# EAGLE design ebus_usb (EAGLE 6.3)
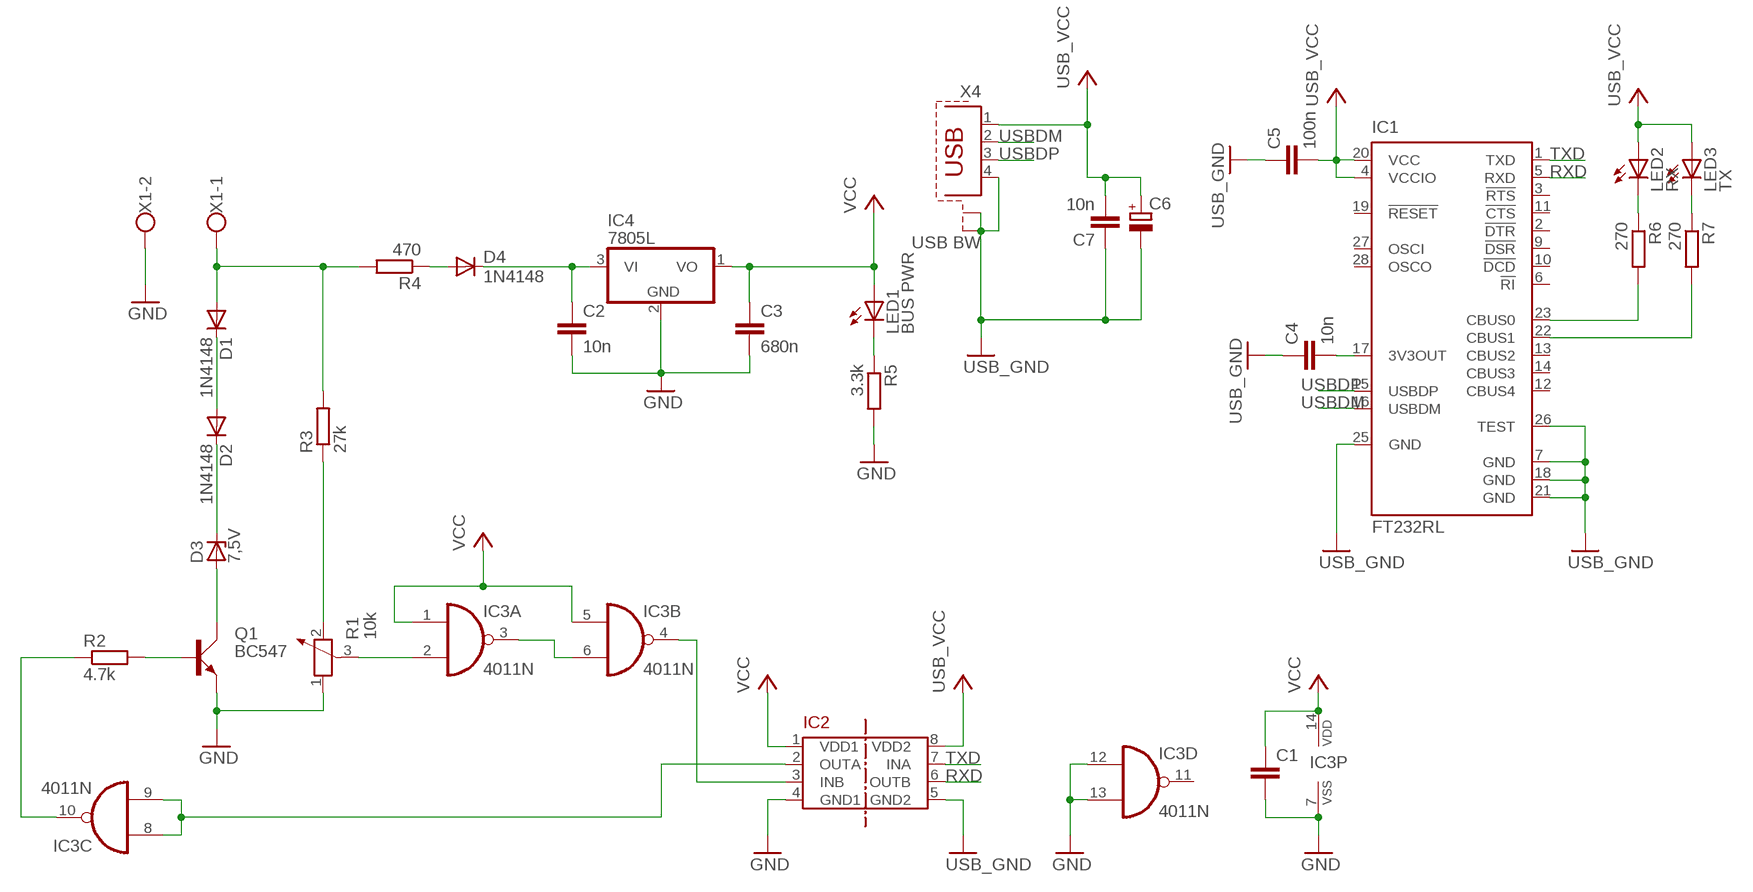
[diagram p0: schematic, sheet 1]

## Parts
C1  C-EUC0805  [C0805]
C2  10n  C-EUC0805  [C0805]
C3  680n  C-EU050-045X075  [C050-045X075]
C4  10n  C-EUC0805  [C0805]
C5  100n  C-EUC0805  [C0805]
C6  CPOL-EUE2.5-6  [E2,5-6]
C7  10n  C-EUC0805  [C0805]
D1  1N4148  1N4148DO35-7  [DO35-7]
D2  1N4148  1N4148DO35-7  [DO35-7]
D3  7,5V  ZENER-DIODEDO34-7  [DO34Z7]
D4  1N4148  1N4148DO35-7  [DO35-7]
IC1  FT232RL  [SSOP28]
IC2  ADUM1201  [SO8]
IC3  4011N  [DIL14]
IC4  7805L  [TO92]
LED1  BUS PWR  LED3MM  [LED3MM]
LED2  RX  LED3MM  [LED3MM]
LED3  TX  LED3MM  [LED3MM]
Q1  BC547  [SOT54A]
R1  10k  POTENTIOMETER_PT-10  [PT-10]
R2  4.7k  R-EU_0204/7  [0204/7]
R3  27k  R-EU_0204/7  [0204/7]
R4  470  R-EU_0204/7  [0204/7]
R5  3.3k  R-EU_0204/7  [0204/7]
R6  270  R-EU_0204/7  [0204/7]
R7  270  R-EU_0204/7  [0204/7]
X1  W237-102  [W237-102]
X4  USB BW  PN61729-S  [PN61729-S]

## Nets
GND: C1.2 C2.2 C3.2 IC2.4(GND1) IC3.7(P:VSS) IC3.12(D:I0) IC3.13(D:I1) IC4.2(GND) Q1.E R1.1 R5.2 X1.2
N$1: D1.A R3.2 R4.2 X1.1
N$2: D1.C D2.A
N$3: D2.C D3.C
N$4: D3.A Q1.C
N$5: D4.A R4.1
N$6: R1.2 R3.1
N$7: Q1.B R2.2
N$8: IC3.10(C:O) R2.1
N$9: IC2.2(OUTA) IC3.8(C:I0) IC3.9(C:I1)
N$10: C2.1 D4.C IC4.3(VI)
N$11: IC1.23(CBUS0) R6.2
N$12: LED1.K(C) R5.1
N$13: IC3.2(A:I1) R1.3
N$14: IC3.3(A:O) IC3.6(B:I1)
N$15: IC2.3(INB) IC3.4(B:O)
N$16: IC1.22(CBUS1) R7.2
N$17: LED2.K(C) R6.1
N$18: LED3.K(C) R7.1
N$19: C4.2 IC1.17(3V3OUT)
RXD: IC1.5(RXD) IC2.6(OUTB)
TXD: IC1.1(TXD) IC2.7(INA)
USB_GND: C4.1 C5.1 C6.- C7.1 IC1.7(GND) IC1.18(GND) IC1.21(GND) IC1.25(GND) IC1.26(TEST) IC2.5(GND2) X4.4 X4.S1 X4.S2
USB_VCC: C5.2 C6.+ C7.2 IC1.4(VCCIO) IC1.20(VCC) IC2.8(VDD2) LED2.A LED3.A X4.1
USBDM: IC1.16(USBDM) X4.2
USBDP: IC1.15(USBDP) X4.3
VCC: C1.1 C3.1 IC2.1(VDD1) IC3.1(A:I0) IC3.5(B:I0) IC3.14(P:VDD) IC4.1(VO) LED1.A
Unconnected: IC1.2(!DTR) IC1.3(!RTS) IC1.6(!RI) IC1.9(!DSR) IC1.10(!DCD) IC1.11(!CTS) IC1.12(CBUS4) IC1.13(CBUS2) IC1.14(CBUS3) IC1.19(!RESET) IC1.27(OSCI) IC1.28(OSCO) IC3.11(D:O)

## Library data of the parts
C1-C5 C7 = rcl:C-EU: CAPACITOR, European symbol
C6 = rcl:CPOL-EU: POLARIZED CAPACITOR, European symbol
D1 D2 D4 = diode:1N4148: DIODE
D3 = diode:ZENER-DIODE: Z-Diode
IC1 = ftdichip:FT232R: Source: http://www.ftdichip.com/Documents/DataSheets/DS_FT232R_v104.pdf; MPN: FT232RL; OC_FARNELL: 1146032; OC_NEWARK: 91K9918
IC2 = Bus-isolators:ADUM1201
IC3 = 40xx:4011: Quad 2-input NAND
IC4 = linear:78*: Positive VOLTAGE REGULATOR Source: http://cache.national.com/ds/LM/LM78L05.pdf http://www.fairchildsemi.com/ds/LM/LM7805.pdf
LED1-LED3 = led:LED: LED
Q1 = transistor-small-signal:BC547: NPN TRANSISTOR
R1 = rcl:POTENTIOMETER_: Potentiometer
R2-R7 = rcl:R-EU_: RESISTOR, European symbol
X1 = con-wago-500:W237-102: WAGO SCREW CLAMP; MPN: 237-102; OC_FARNELL: unknown; OC_NEWARK: 70K9898
X4 = con-berg:PN61729-S: BERG USB connector; OC_FARNELL: unknown; OC_NEWARK: unknown

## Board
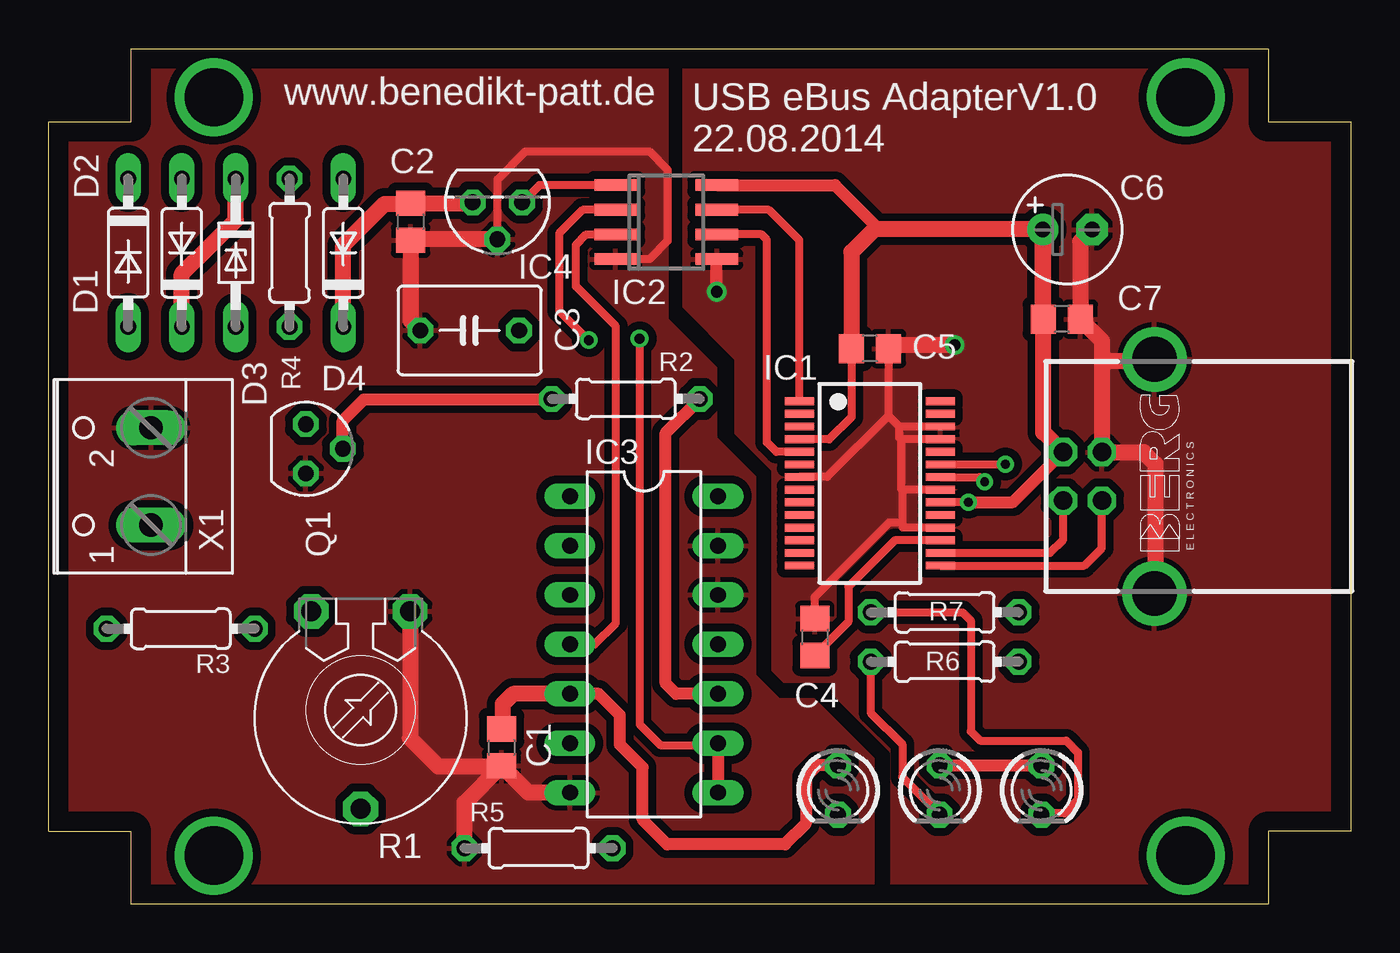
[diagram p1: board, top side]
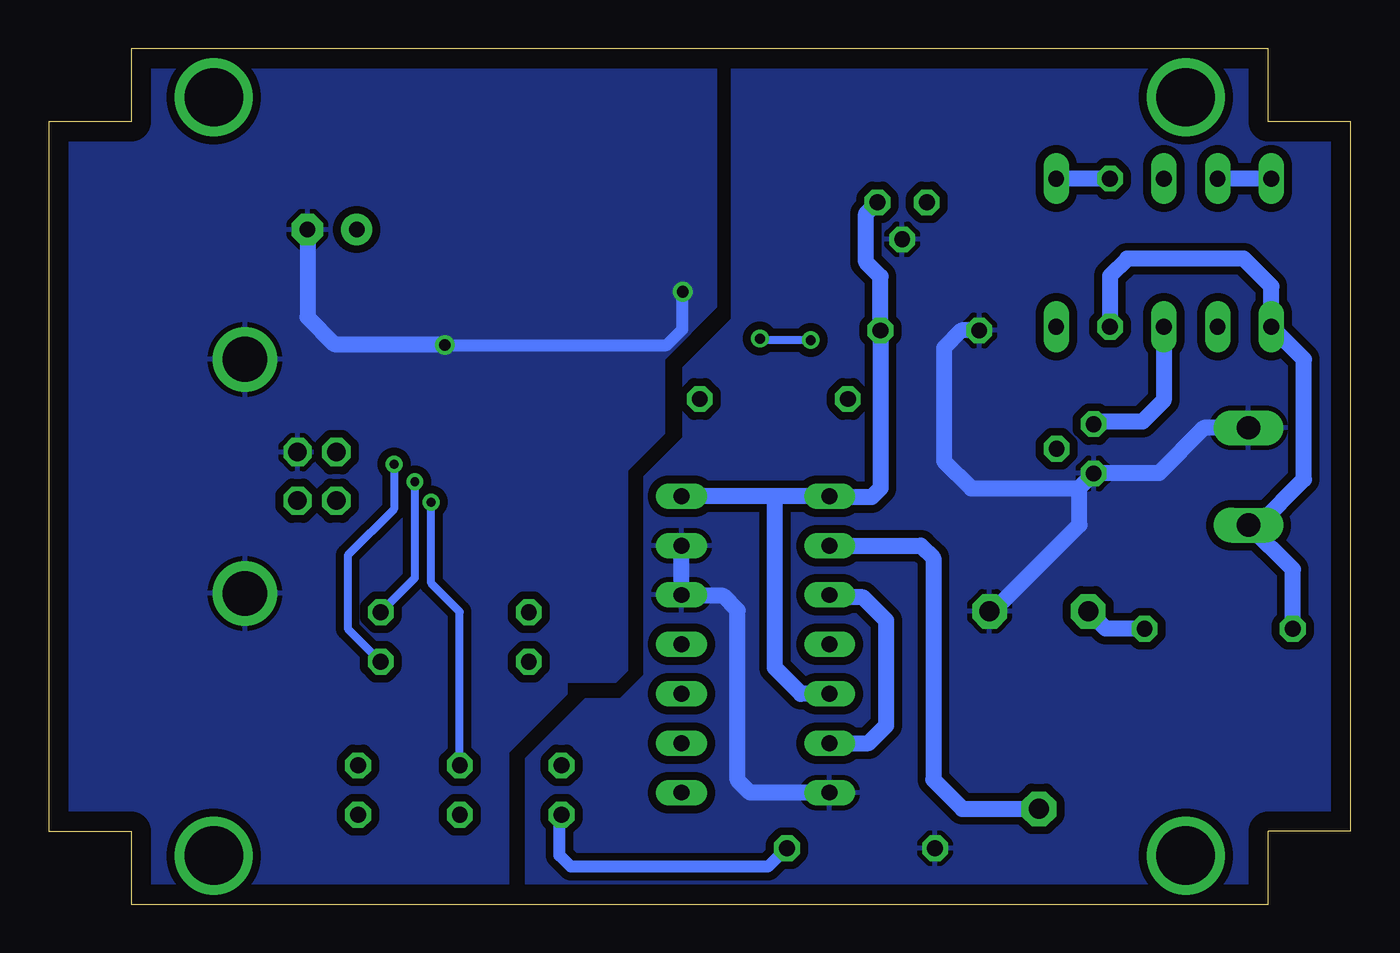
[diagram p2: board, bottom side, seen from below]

Size 67 x 44 mm. Coordinates in mm from the lower left corner, seen from the top.
Outline: 0,3.75 0,40.25 4.25,40.25 4.25,44 62.75,44 62.75,40.25 67,40.25 67,3.75 62.75,3.75 62.75,0 4.25,0 4.25,3.75 0,3.75
Copper layers (1*16): Top 0.035mm / dielectric 1.5mm / Bottom 0.035mm
Design rules "default": minimum track width 10mil, minimum drill 24mil, track to track 8mil, track to pad 8mil, pad to pad 8mil, via to via 8mil, smd to smd 8mil, copper to edge 40mil, drill to drill 8mil, minimum pad ring 10mil, minimum via ring 8mil, stop-mask expansion 4mil, vias tented up to drill 0mil, thermal gap 10mil

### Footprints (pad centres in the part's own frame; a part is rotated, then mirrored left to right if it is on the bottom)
C0805 = smd 1.3 x 1.5: 1 -0.95,0; 2 0.95,0
C050-045X075 = drill 0.813 octagon: 1 -2.54,0; 2 2.54,0
E2,5-6 = drill 0.813 pad 1.6: + -1.27,0 | drill 0.813 pad 1.6 octagon: - 1.27,0
DO35-7 = drill 0.813 long: A 3.81,0; C -3.81,0
DO34Z7 = drill 0.813 long: A 3.81,0; C -3.81,0
SSOP28 = smd 0.4 x 1.5: 1 -4.225,-3.625; 2 -3.575,-3.625; 3 -2.925,-3.625; 4 -2.275,-3.625; 5 -1.625,-3.625; 6 -0.975,-3.625; 7 -0.325,-3.625; 8 0.325,-3.625; 9 0.975,-3.625; 10 1.625,-3.625; 11 2.275,-3.625; 12 2.925,-3.625; 13 3.575,-3.625; 14 4.225,-3.625; 15 4.225,3.625; 16 3.575,3.625; 17 2.925,3.625; 18 2.275,3.625; 19 1.625,3.625; 20 0.975,3.625; 21 0.325,3.625; 22 -0.325,3.625; 23 -0.975,3.625; 24 -1.625,3.625; 25 -2.275,3.625; 26 -2.925,3.625; 27 -3.575,3.625; 28 -4.225,3.625
SO8 = smd 0.6 x 2.2: 1 -1.905,-2.6; 2 -0.635,-2.6; 3 0.635,-2.6; 4 1.905,-2.6; 5 1.905,2.6; 6 0.635,2.6; 7 -0.635,2.6; 8 -1.905,2.6
DIL14 = drill 0.813 long: 1 -7.62,-3.81; 2 -5.08,-3.81; 3 -2.54,-3.81; 4 0,-3.81; 5 2.54,-3.81; 6 5.08,-3.81; 7 7.62,-3.81; 8 7.62,3.81; 9 5.08,3.81; 10 2.54,3.81; 11 0,3.81; 12 -2.54,3.81; 13 -5.08,3.81; 14 -7.62,3.81
TO92 = drill 0.813 octagon: 1 -1.27,0; 2 0,1.905; 3 1.27,0
LED3MM = drill 0.813 octagon: A -1.27,0; K 1.27,0
SOT54A = drill 0.813 octagon: B 0,1.905; C -1.27,0; E 1.27,0
PT-10 = drill 1.016 pad 1.778 octagon: 1 -2.54,-5.08; 2 2.54,-5.08; 3 0,5.08
0204/7 = drill 0.813 octagon: 1 -3.81,0; 2 3.81,0
W237-102 = drill 1.194 long: 1 -2.5,-1.27; 2 2.5,-1.27
PN61729-S = drill 0.95 octagon: 1 1.25,4.71; 2 -1.25,4.71; 3 -1.25,2.71; 4 1.25,2.71 | drill 2.3 pad 2.9: S1 -6.02,0; S2 6.02,0

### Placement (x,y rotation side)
C1  23.31,8.06 270 top
C2  18.63,35.1 270 top
C3  21.66,29.5 180 top
C4  39.42,13.74 270 top
C5  42.26,28.57 180 top
C6  52.41,34.7 0 top
C7  52.13,30.09 180 top
D1  4.09,33.5 270 top
D2  6.86,33.5 90 top
D3  9.63,33.5 270 top
D4  15.16,33.5 90 top
IC1  42.25,21.64 270 top
IC2  31.78,35.08 270 top
IC3  30.63,13.36 270 top
IC4  23.09,36.09 180 top
LED1  40.61,5.87 270 top
LED2  45.85,5.87 270 top
LED3  51.08,5.87 270 top
Q1  13.23,23.42 270 top
R1  16.05,9.98 180 top
R2  29.69,25.98 180 top
R3  6.8,14.16 180 top
R4  12.4,33.5 270 top
R5  25.2,2.88 180 top
R6  46.1,12.47 0 top
R7  46.1,15.01 0 top
X1  4,22 90 top
X4  56.9,22 90 top

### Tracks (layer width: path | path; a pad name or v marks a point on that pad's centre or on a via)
GND
  Top 0.406: IC4.2 23.09,37.26 24.54,38.71 30.91,38.71 31.85,37.77 31.85,34.11 30.91,33.17 IC2.4
  Top 0.813: IC4.2 18.67,34.19 C2.2 18.63,30 C3.2 | R1.1 18.59,8.53 20.04,7.09 23.28,7.09 C1.2 | IC3.7 24.68,5.74 C1.2 | R5.2 21.39,5.2 C1.2
  Bottom 0.813: X1.2 7.55,24.5 9.88,22.17 13.21,22.17 Q1.E 13.99,21.39 | C3.2 20.03,29.5 20.93,28.6 20.93,22.78 19.53,21.39 13.99,21.39 | R1.1 18.41,15.06 13.97,19.51 13.97,21.36 13.99,21.39 | IC3.7 30.91,5.74 31.55,6.38 31.55,15.11 32.28,15.85 34.39,15.85 IC3.12 IC3.13
  pour Bottom (isolate 0.406): 0,40.2 4.3,40.2 4.3,44 31.9,44 31.9,30.1 34.4,27.6 34.4,24 36.4,22 36.4,11.8 37.6,10.6 39.4,10.6 42.5,7.5 42.5,0 4.3,0 4.3,3.8 0,3.8
  pour Top (isolate 0.406): 0,40.2 4.3,40.2 4.3,44 31.9,44 31.9,30.1 34.4,27.6 34.4,24 36.4,22 36.4,11.8 37.6,10.6 39.4,10.6 42.5,7.5 42.5,0 4.3,0 4.3,3.8 0,3.8
N$1
  Bottom 0.813: R4.2 12.39,32.31 11.51,33.2 5.51,33.2 4.09,31.77 D1.A 2.41,28.02 2.41,21.84 4.76,19.5 X1.1 2.99,17.22 R3.2
N$2
  Bottom 0.813: D1.C D2.A
N$3
  Top 0.813: D2.C 6.86,32.41 8.18,33.73 9.63,35.18 D3.C
N$4
  Bottom 0.813: D3.A 9.63,25.91 10.72,24.82 13.11,24.82 Q1.C
N$5
  Bottom 0.813: R4.1 D4.A
N$6
  Bottom 0.813: R3.1 12.62,14.16 R1.2
N$7
  Top 0.61: Q1.B 15.14,24.87 16.23,25.96 25.86,25.96 R2.2
N$8
  Top 0.61: IC3.10 32.28,10.82 31.75,11.35 31.75,24.23 R2.1
N$9  (via drill 0.5)
  Top 0.406: IC2.2 27.48,35.71 26.26,34.49 26.26,30.53 v27.79,29.01 | v30.4,29.08 30.4,9.25 31.47,8.18 34.34,8.18 IC3.9
  Top 0.61: IC3.9 IC3.8
  Bottom 0.406: v27.79,29.01 30.33,29.01 v30.4,29.08
N$10
  Top 0.813: D4.C 15.16,33.88 17.3,36.02 18.59,36.02 C2.1 21.77,36.05 IC4.3
N$11  (via drill 0.46)
  Top 0.406: IC1.23 49.21,22.61 v49.23,22.63
  Bottom 0.406: v49.23,22.63 49.23,20.32 51.61,17.93 51.61,14.17 R6.2
N$12
  Bottom 0.61: R5.1 29.05,2.88 30,1.93 40.13,1.93 40.72,2.52 40.72,4.5 LED1.K
N$13
  Bottom 0.813: IC3.2 22.12,18.44 21.49,17.8 21.49,6.4 19.99,4.9 R1.3
N$14
  Bottom 0.813: IC3.6 24.82,8.28 23.9,9.2 23.9,14.58 25.09,15.77 26.7,15.77 IC3.3
N$15
  Top 0.406: IC3.4 28.09,13.36 29.18,14.45 29.18,29.72 27.13,31.77 27.13,33.91 27.66,34.44 IC2.3
N$16  (via drill 0.46)
  Top 0.406: IC1.22 47.91,21.96 v48.16,21.72
  Bottom 0.406: v48.16,21.72 48.16,16.76 R7.2
N$17
  Top 0.406: R6.1 42.29,9.86 43.92,8.23 43.92,6.53 LED2.K
N$18
  Top 0.406: R7.1 47.02,15.01 47.45,14.58 47.45,8.89 47.93,8.41 52.35,8.41 52.96,7.8 52.96,5.36 52.27,4.67 51.16,4.67 LED3.K
N$19
  Top 0.406: IC1.17 43.53,18.71 41.15,16.33 41.15,14.52 C4.2
N$20  (via drill 3)
  other vias: 58.5,41.5
N$21  (via drill 3)
  other vias: 58.5,2.5
N$22  (via drill 3)
  other vias: 8.5,41.5
N$23  (via drill 3)
  other vias: 8.5,2.5
RXD
  Top 0.406: IC1.5 37.44,23.27 36.96,23.75 36.96,34.16 36.68,34.44 IC2.6
TXD
  Top 0.406: IC1.1 38.62,34.15 37.06,35.71 IC2.7
USB_GND  (via drill 0.6)
  Top 0.406: C5.1 43.21,25.12 | 43.21,25.12 40.06,21.97 IC1.7 | IC1.26 43.77,24.57 | 43.77,24.57 43.21,25.12 | IC1.25 43.85,23.91 | 43.85,23.91 43.76,24 43.76,24.56 43.77,24.57 | IC1.21 43.91,21.32 | 43.91,21.32 43.87,21.36 43.87,23.9 43.85,23.91 | IC1.18 43.96,19.36 43.94,19.38 43.94,19.63 | 43.94,19.63 43.94,21.29 43.91,21.32 | C4.1 39.42,15.8 43.26,19.63 43.94,19.63
  Top 0.61: v34.37,31.5 34.37,33.16 IC2.5
  Top 0.813: C6.- 53.08,34.09 C7.1 54.19,28.97 54.19,27.91 | 54.19,27.91 X4.4 56.33,23.25 56.95,22.63 56.95,16.03 X4.S1 | X4.S2 56.8,27.91 54.19,27.91 | v46.61,28.75 43.39,28.75 C5.1
  Bottom 0.61: v46.61,28.75 35.2,28.75 34.39,29.57 34.39,31.47 v34.37,31.5
  Bottom 0.813: C6.- 53.68,30.19 52.3,28.8 46.66,28.8 v46.61,28.75
  pour Bottom (isolate 0.406): 32.6,44 62.7,44 62.7,40.2 67,40.2 67,3.8 62.8,3.8 62.8,0 43.3,0 43.3,7.8 40.3,10.8 40.3,11.4 37.8,11.4 37.2,12 37.2,22.3 35.3,24.2 35.3,28 32.6,30.7
  pour Top (isolate 0.406): 62.7,44 62.7,40.2 67,40.2 67,3.8 62.8,3.8 62.8,0 43.3,0 43.3,7.8 40.3,10.8 40.3,11.4 37.8,11.4 37.2,12 37.2,22.3 35.3,24.2 35.3,28 32.6,30.7 32.6,44 62.7,44
USB_VCC  (via drill 0.46)
  Top 0.406: C5.2 41.31,25.05 40.16,23.9 38.64,23.9 IC1.4 | v47.32,20.68 45.89,20.68 IC1.20
  Top 0.61: IC2.8 40.46,36.98 42.72,34.72 | LED2.A LED3.A | v47.32,20.68 49.62,20.68 X4.1
  Top 0.813: X4.1 51.18,24.26 | 51.18,24.26 C7.2 51.14,30.12 C6.+ | 51.18,24.26 51.18,34.67 51.13,34.72 42.72,34.72 42.49,34.72 41.3,33.53 C5.2
  Bottom 0.406: LED2.A 45.85,15.04 47.32,16.51 v47.32,20.68
USBDM
  Top 0.406: IC1.16 51.52,18.07 52.2,18.75 X4.2
USBDP
  Top 0.406: IC1.15 53.28,17.41 54.18,18.31 54.18,20.74 X4.3
VCC
  Top 0.406: IC2.1 25.25,36.98 IC4.1
  Top 0.61: LED1.A 39.55,7.14 38.96,6.55 38.96,4.14 37.9,3.07 31.83,3.07 30.56,4.34 30.56,7.04 29.39,8.2 29.39,9.73 28.3,10.82 IC3.5
  Top 0.813: IC3.5 23.9,10.82 23.37,10.29 23.37,9.08 C1.1
  Bottom 0.813: IC4.1 24.94,35.51 24.94,33.02 24.2,32.28 C3.1 24.2,21.39 24.66,20.93 26.77,20.93 IC3.1 29.54,20.98 | 29.54,20.98 IC3.14 | IC3.5 28.3,10.82 29.64,12.17 29.64,20.88 29.54,20.98

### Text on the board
tNames: www.benedikt-patt.de | USB eBus AdapterV1.0 / 22.08.2014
